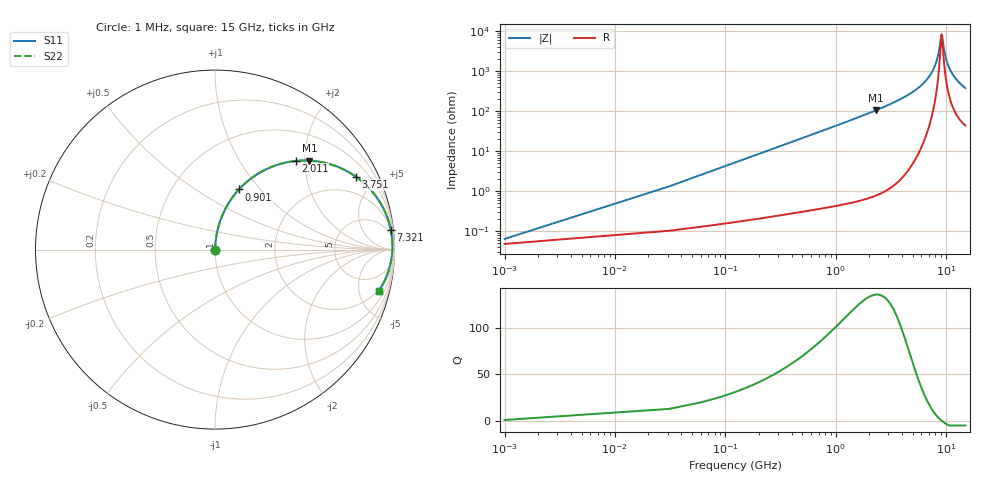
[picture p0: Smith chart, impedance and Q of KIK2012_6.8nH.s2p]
!version-2
!date-01.2022
!Series
# MHz S RI R 50
!Freq ReS11 ImS11 ReS21 ImS21 ReS12 ImS12 ReS22 ImS22
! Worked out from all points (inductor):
!   501 points, 1 MHz to 15 GHz, reference 50 ohm
!   read as one part in series: L = 6.8 nH near 61 MHz
!   highest Q = 136 at 2.311 GHz (marker M1), where L = 7.26 nH
!   self-resonance near 9.121 GHz
!   S11 on the Smith chart (normalised r, x): 1 MHz: 1.00, +0.00; 901 MHz: 1.01, +0.78; 2.011 GHz: 1.01, +1.81; 3.751 GHz: 1.04, +3.85; 7.321 GHz: 2, +17; 15 GHz: 1.88, -7.52
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1  0.000484 0.000427  0.9995 -0.000427  0.9995 -0.000427  0.000484 0.000427
91  0.00301 0.0387  0.997 -0.0387  0.997 -0.0387  0.00301 0.0387
181  0.0079 0.0766  0.9921 -0.0766  0.9921 -0.0766  0.0079 0.0766
301  0.0186 0.126  0.9814 -0.126  0.9814 -0.126  0.0186 0.126
451  0.0386 0.1852  0.9614 -0.1852  0.9614 -0.1852  0.0386 0.1852
901  0.1339 0.3353  0.8661 -0.3353  0.8661 -0.3353  0.1339 0.3353
1381  0.2689 0.4392  0.7311 -0.4392  0.7311 -0.4392  0.2689 0.4392
2011  0.4495 0.4937  0.5505 -0.4937  0.5505 -0.4937  0.4495 0.4937
2311  0.5265 0.4956  0.4735 -0.4956  0.4735 -0.4956  0.5265 0.4956
2521  0.5756 0.4906  0.4244 -0.4906  0.4244 -0.4906  0.5756 0.4906
3751  0.7857 0.4057  0.2143 -0.4057  0.2143 -0.4057  0.7857 0.4057
5011  0.8997 0.2924  0.1003 -0.2924  0.1003 -0.2924  0.8997 0.2924
7321  0.9791 0.1114  0.0209 -0.1114  0.0209 -0.1114  0.9791 0.1114
7501  0.9814 0.0993  0.0186 -0.0993  0.0186 -0.0993  0.9814 0.0993
8401  0.9879 0.0425  0.0121 -0.0425  0.0121 -0.0425  0.9879 0.0425
9121  0.9882 0.0014  0.0118 -0.0014  0.0118 -0.0014  0.9882 0.0014
9241  0.9879 -0.00512  0.0121 0.00512  0.0121 0.00512  0.9879 -0.00512
9691  0.986 -0.0287  0.014 0.0287  0.014 0.0287  0.986 -0.0287
10021  0.9839 -0.0453  0.0161 0.0453  0.0161 0.0453  0.9839 -0.0453
11011  0.9749 -0.0913  0.0251 0.0913  0.0251 0.0913  0.9749 -0.0913
12511  0.9548 -0.1517  0.0452 0.1517  0.0452 0.1517  0.9548 -0.1517
15000  0.9113 -0.2319  0.0887 0.2319  0.0887 0.2319  0.9113 -0.2319
